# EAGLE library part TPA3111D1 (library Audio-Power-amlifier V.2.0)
10-W FILTER-FREE MONO CLASS-D AUDIO POWER AMPLIFIER with SPEAKER GUARnd
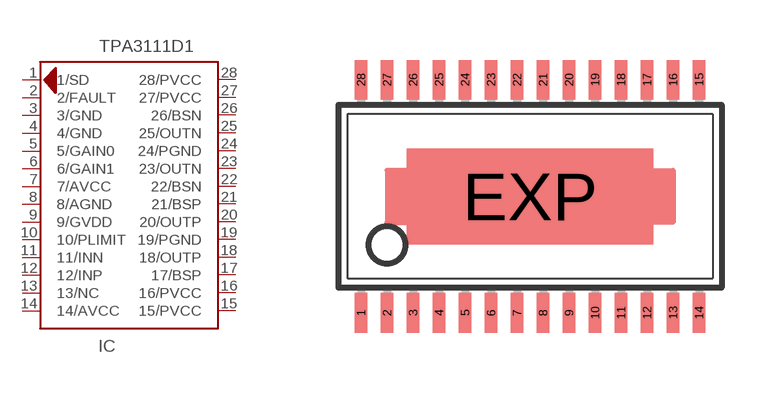
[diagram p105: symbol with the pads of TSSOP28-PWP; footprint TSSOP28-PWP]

Designator prefix IC

## TPA3111D1  [TSSOP28-PWP]
1  1/SD  out
2  2/FAULT  out
3  3/GND  pwr
4  4/GND  pwr
5  5/GAIN0
6  6/GAIN1
7  7/AVCC  pwr
8  8/AGND  pwr
9  9/GVDD  out
10  10/PLIMIT  in
11  11/INN  in
12  12/INP  in
13  13/NC  nc
14  14/AVCC  pwr
15  15/PVCC  pwr
16  16/PVCC  pwr
17  17/BSP  in
18  18/OUTP  out
19  19/PGND  pwr
20  20/OUTP  out
21  21/BSP  in
22  22/BSN  in
23  23/OUTN  out
24  24/PGND  pwr
25  25/OUTN  out
26  26/BSN  in
27  27/PVCC  pwr
28  28/PVCC  pwr

## Footprint TSSOP28-PWP (pad centres in mm)
Power Thin Shrink Small Outline Plastic 28
smd 0.305 x 0.991: 1 -4.225,-2.918; 2 -3.575,-2.918; 3 -2.925,-2.918; 4 -2.275,-2.918; 5 -1.625,-2.918; 6 -0.975,-2.918; 7 -0.325,-2.918; 8 0.325,-2.918; 9 0.975,-2.918; 10 1.625,-2.918; 11 2.275,-2.918; 12 2.925,-2.918; 13 3.575,-2.918; 14 4.225,-2.918; 15 4.225,2.918; 16 3.575,2.918; 17 2.925,2.918; 18 2.275,2.918; 19 1.625,2.918; 20 0.975,2.918; 21 0.325,2.918; 22 -0.325,2.918; 23 -0.975,2.918; 24 -1.625,2.918; 25 -2.275,2.918; 26 -2.925,2.918; 27 -3.575,2.918; 28 -4.225,2.918
smd 6.17 x 2.4: EXP 0,0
